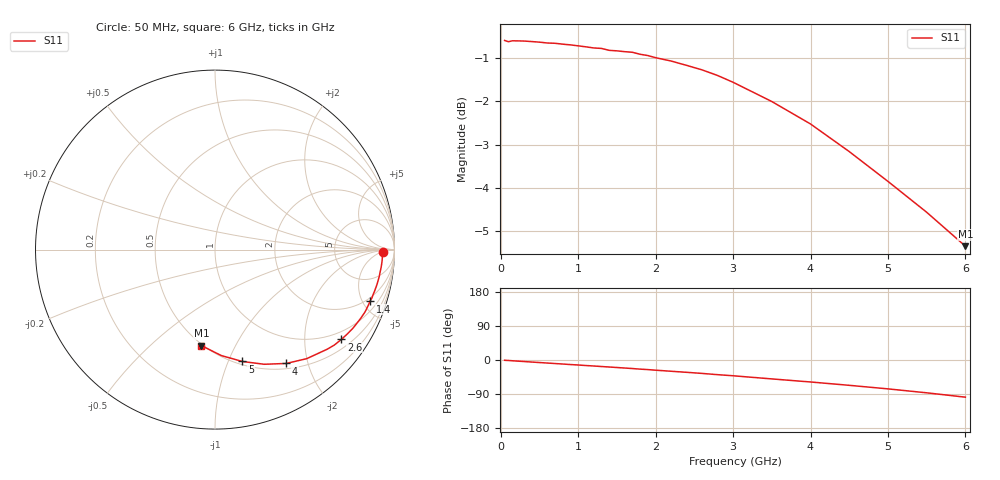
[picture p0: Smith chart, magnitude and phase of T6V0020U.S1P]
! SIEMENS Discrete & RF Semiconductors
! BAT62
! Si Schottky Diode in SOT143
! IF = 0.02 mA
! S-Parameters:  February  1997
# GHz  S  MA  R  50
!  f  S11
! GHz  MAG  ANG
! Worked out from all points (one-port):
!   34 points, 50 MHz to 6 GHz, reference 50 ohm
!   lowest |S11| = -5.3 dB at 6 GHz (marker M1), VSWR 3.35, Z = 24.5 - j37 ohm
!   |S11| at or under -10 dB: nowhere
!   S11 on the Smith chart (normalised r, x): 50 MHz: 29, -5; 1.4 GHz: 1.68, -5.65; 2.6 GHz: 0.75, -2.96; 4 GHz: 0.57, -1.65; 5 GHz: 0.53, -1.13; 6 GHz: 0.49, -0.74
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0.05  0.9344 -0.7
0.1  0.9313 -1.3
0.15  0.9335 -2.0
0.4  0.9316 -5.4
0.7  0.9274 -9.3
0.8  0.9252 -10.6
0.9  0.9234 -12.0
1  0.9211 -13.2
1.1  0.9186 -14.6
1.2  0.9159 -15.8
1.3  0.9148 -17.2
1.4  0.9101 -18.5
1.6  0.9069 -21.2
1.7  0.9054 -22.5
1.8  0.9006 -24.1
1.9  0.8975 -25.3
2  0.8925 -26.9
2.2  0.8846 -29.7
2.4  0.8744 -32.5
2.6  0.864 -35.4
2.8  0.8511 -38.7
3  0.8359 -41.6
3.5  0.7942 -49.9
4  0.748 -58.0
4.5  0.695 -66.8
5  0.642 -76.2
5.5  0.5913 -86.6
6  0.5402 -98.1
